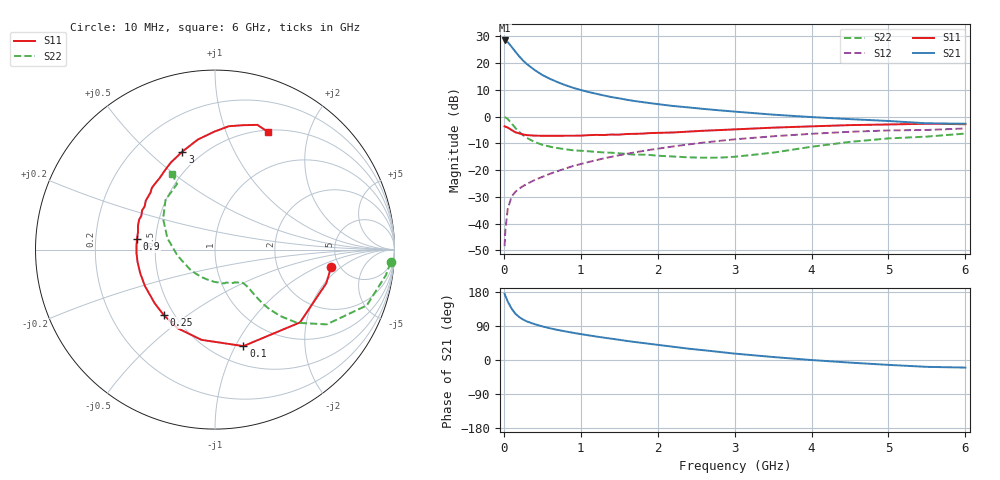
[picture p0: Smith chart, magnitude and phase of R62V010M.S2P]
! SIEMENS Small Signal Semiconductors
! BFR193
! Si NPN RF Bipolar Junction Transistor in SOT23
! VCE = 2 V  IC = 10 mA
! Common Emitter S-Parameters:  May  1996
# GHz  S  MA  R  50
!  f  S11  S21  S12  S22
! GHz  MAG  ANG  MAG  ANG  MAG  ANG  MAG  ANG
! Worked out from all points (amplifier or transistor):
!   36 points, 10 MHz to 6 GHz, reference 50 ohm
!   highest |S21| = 28.4 dB at 10 MHz (marker M1)
!   |S21| within 3 dB of that: start of sweep to 118 MHz
!   unconditionally stable (mu >= 1): 716.1 MHz to 2.001 GHz
!   at 250 MHz: K = 0.65, MSG = 23.4 dB, |S12| = -26.0 dB
!   at 1.4 GHz: K = 1.04, MAG = 10.0 dB, |S12| = -15.0 dB
!   at 6 GHz: K = 0.95, MSG = 0.9 dB, |S12| = -4.5 dB
!   lowest NFmin = 1.30 dB at 450 MHz
!   S11 on the Smith chart (normalised r, x): 10 MHz: 4.26, -1.48; 100 MHz: 0.69, -1.08; 250 MHz: 0.44, -0.41; 900 MHz: 0.39, +0.06; 3 GHz: 0.39, +0.64; 6 GHz: 0.52, +1.42
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0.01  0.6549 -8.7  26.34 174.8  0.0038 86.0  0.9807 -4.2
0.02  0.6473 -17.0  26.29 169.2  0.0077 82.9  0.9629 -8.5
0.05  0.6236 -40.6  24.56 154.7  0.0185 73.9  0.9009 -20.2
0.1  0.5605 -73.6  20.15 135.8  0.0319 62.1  0.7488 -33.8
0.15  0.5084 -98.5  16.25 122.1  0.0393 56.5  0.6116 -41.8
0.2  0.4851 -115.5  13.29 113.3  0.0451 55.0  0.5165 -45.6
0.25  0.4629 -128.2  11.1 106.8  0.0504 54.5  0.4482 -47.6
0.3  0.4499 -138.3  9.538 101.7  0.0551 55.8  0.3986 -48.6
0.4  0.4401 -152.5  7.393 94.6  0.0652 57.8  0.3347 -48.9
0.5  0.4369 -162.3  5.974 88.7  0.0746 58.8  0.2974 -48.7
0.6  0.4369 -170.6  5.053 83.7  0.0854 60.2  0.2742 -48.9
0.7  0.4378 -177.0  4.384 79.3  0.0959 61.6  0.2575 -49.3
0.9  0.4386 172.3  3.443 71.8  0.1191 62.5  0.2344 -51.0
1.1  0.4491 162.9  2.875 65.1  0.1416 62.4  0.2248 -54.7
1.3  0.4515 155.3  2.475 59.0  0.1655 61.6  0.2136 -58.9
1.6  0.4725 144.7  2.055 50.3  0.2017 59.4  0.1995 -67.9
2.2  0.5042 127.6  1.575 35.0  0.2764 53.4  0.1795 -91.7
3  0.5757 108.4  1.237 16.9  0.3755 42.4  0.1773 -140.0
3.5  0.6203 98.9  1.085 7.9  0.4282 34.6  0.2117 -170.8
4.5  0.6917 83.6  0.895 -6.9  0.5194 19.7  0.3364 149.3
5.5  0.7341 71.2  0.747 -18.1  0.5618 4.3  0.4222 120.1
6  0.7187 65.7  0.735 -20.0  0.5991 -0.2  0.4813 119.6
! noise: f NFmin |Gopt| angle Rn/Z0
0.45  1.3  0.22  143  0.11
0.9  1.3  0.34  160  0.11
1.8  2.05  0.54  -153  0.14
